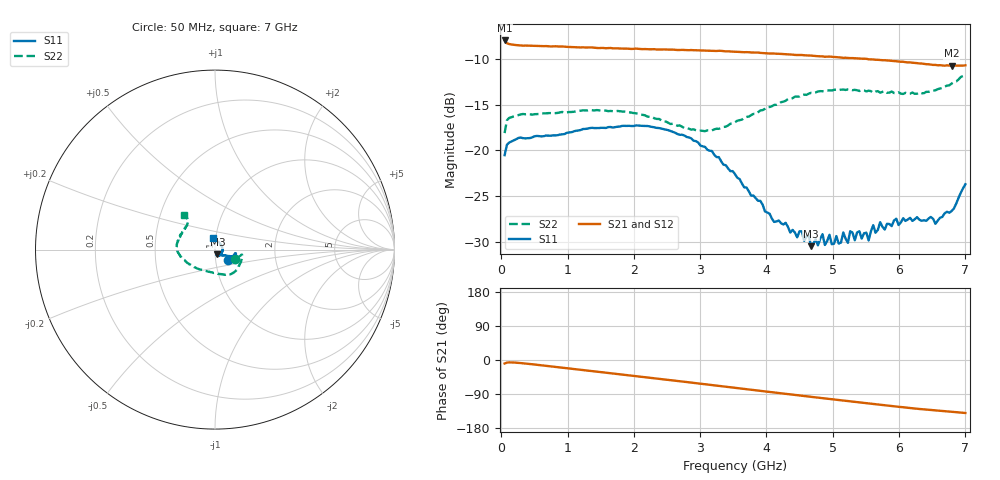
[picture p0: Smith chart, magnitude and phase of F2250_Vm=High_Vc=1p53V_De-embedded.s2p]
! Integrated Device Technology
! Corporate Headquarters
! 6024 Silver Creek Valley Road
! San Jose, CA 95138  USA
! Phone:  1-408-284-8200
! Toll Free:  1-800-223-1366
! Webpage:  http://www.idt.com/
! Timing and RF Division
! 515 Groton Road, Suite 102
! Westford, MA 01886-6024
! Device:  F2250
! Description: Voltage Variable RF Attenuator
! Frequency:  50.0 -  6000.00 MHz
! Package:  3x3 mm Thin QFN Plastic Package: 16 pin
! Ports:  2 RF, 3 DC
!  Pin  1  = GND
!  Pin  2  = NC
!  Pin  3  = RF1  = Port 1
!  Pin  4  = NC
!  Pin  5  = GND
!  Pin  6  = GND
!  Pin  7  = GND
!  Pin  8  = GND
!  Pin  9  = NC
!  Pin 10  = RF2  = Port 2
!  Pin 11  = NC
!  Pin 12  = GND
!  Pin 13  = GND
!  Pin 14  = VCNTRL
!  Pin 15  = VDD
!  Pin 16  = VMODE
! Vcntrl:  1.530 Volts
! Vmode:  +3.300 Volts
! Vdd:  +3.30  Volts
! Current:  1.329 mA
! Data:  The device was measured on a the F2250 evaluation board which has
!  individual transmission lines to the RF pins.  Data was collected
!  using a calibrated network analyzer.  The evaluation board was
!  de-embedded using a TRL calibration technique.
!  The reference plane is the edge of the package pin.
! Misc:  SN 10
!  Action Tracker AT0258
! Date Measured:  2014-11-26
! Date:  2015-10-15  MJV
! Note:
!  Integrated Device Technology supplies this data as a sample of measured
!  data at the package pin for this product.  Your particular data for this
!  product may vary.
!  Data was taken at 25 degrees C.
!  Integrated Device Technology reserves the right to change this data at anytime.
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# GHz S dB R 50
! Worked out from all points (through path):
!   201 points, 50 MHz to 7 GHz, reference 50 ohm
!   highest |S21| = -7.99 dB at 50 MHz (marker M1); lowest = -10.8 dB at 6.792 GHz (marker M2)
!   group delay of S21, straight-line fit = 55.9 ps
!   lowest |S11| = -30.5 dB at 4.672 GHz (marker M3), VSWR 1.06, Z = 51.2 - j2.77 ohm
!   |S11| at or under -10 dB: start of sweep to end of sweep
!   |S22| runs from -18.1 to -11.7 dB; largest |S21 - S12| = 0.0016
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0.05  -20.52 -38.5  -7.99 -9.2  -7.99 -9.2  -18.11 -24.5
0.22375  -18.78 -10.6  -8.50 -7.0  -8.48 -7.0  -16.19 -12.0
1.2315  -17.66 -22.3  -8.74 -26.6  -8.75 -26.6  -15.62 -42.4
2.37825  -17.56 -22.5  -8.98 -49.5  -9.00 -49.6  -16.56 -70.7
2.969  -19.13 -21.1  -9.07 -61.8  -9.06 -61.8  -17.87 -97.9
3.525  -22.59 -27.2  -9.23 -73.4  -9.22 -73.5  -16.92 -131.7
4.11575  -27.81 -48.8  -9.42 -85.7  -9.43 -85.7  -15.03 -158.4
4.67175  -30.46 -64.2  -9.64 -97.2  -9.66 -97.2  -13.71 -174.6
4.7065  -30.18 -70.9  -9.67 -97.9  -9.67 -97.9  -13.73 -175.3
4.8455  -29.14 -67.1  -9.73 -100.7  -9.75 -100.6  -13.54 -178.4
4.88025  -30.32 -64.9  -9.77 -101.3  -9.76 -101.4  -13.51 -179.6
4.94975  -29.21 -67.0  -9.75 -102.8  -9.76 -102.8  -13.45 178.9
5.08875  -30.17 -61.6  -9.83 -105.6  -9.84 -105.7  -13.41 175.5
5.15825  -28.95 -62.6  -9.89 -106.9  -9.89 -107.0  -13.35 174.1
5.22775  -30.10 -61.1  -9.90 -108.4  -9.89 -108.4  -13.33 172.3
5.2625  -28.82 -58.8  -9.92 -109.0  -9.92 -109.1  -13.35 171.8
5.5405  -29.83 -42.3  -10.05 -114.6  -10.04 -114.7  -13.48 164.1
5.61  -28.17 -38.4  -10.07 -116.0  -10.07 -116.0  -13.71 162.8
5.85325  -28.04 -26.1  -10.19 -120.7  -10.21 -120.8  -13.69 155.5
6.54825  -28.02 37.7  -10.66 -133.2  -10.65 -133.3  -13.43 135.2
6.7915  -26.62 70.3  -10.75 -136.5  -10.75 -136.7  -12.70 131.6
7  -23.69 102.1  -10.71 -139.8  -10.72 -139.9  -11.68 131.5
